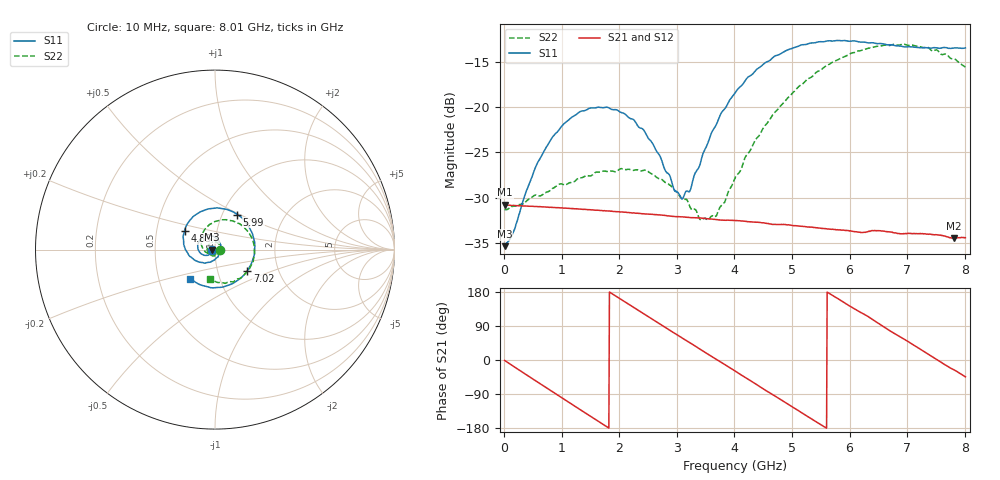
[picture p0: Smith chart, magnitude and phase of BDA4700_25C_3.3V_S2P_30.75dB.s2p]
!Agilent Technologies,E5071B,MY42404982,A.09.10
!Date: Mon Oct 20 18:16:00 2025
!Data & Calibration Information:
!Freq	S11:SOLT2(ON)	S21:SOLT2(ON)	S12:SOLT2(ON)	S22:SOLT2(ON)
# Hz S RI R 50
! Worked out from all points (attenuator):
!   801 points, 10 MHz to 8.01 GHz, reference 50 ohm
!   highest |S21| = -30.79 dB at 20 MHz (marker M1); lowest = -34.5 dB at 7.81 GHz (marker M2)
!   lowest |S11| = -35.4 dB at 10 MHz (marker M3), VSWR 1.03, Z = 48.3 - j0.0984 ohm
!   |S11| at or under -10 dB: start of sweep to end of sweep
!   |S22| runs from -32.5 to -13.0 dB; largest |S21 - S12| = 0.00036
!   S11 on the Smith chart (normalised r, x): 10 MHz: 0.97, -0.00; 4.83 GHz: 0.70, +0.15; 5.99 GHz: 1.17, +0.48; 7.02 GHz: 1.39, -0.35; 8.01 GHz: 0.72, -0.25
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1e7  -0.017 -0.00102  0.0289 -0.00063  0.0288 -0.000637  0.0272 -0.000751
2e7  -0.0174 -0.00161  0.0289 -0.00107  0.0288 -0.00118  0.0271 -0.00109
1.6e8  -0.0178 -0.00977  0.0275 -0.00803  0.0275 -0.00802  0.0273 -0.00773
5.3e8  -0.0346 -0.029  0.017 -0.0226  0.017 -0.0226  0.0168 -0.028
7.3e8  -0.0502 -0.0326  0.0083 -0.0268  0.00832 -0.0268  0.00416 -0.0336
1.35e9  -0.0952 0.00416  -0.0189 -0.0197  -0.0189 -0.0198  -0.0364 -0.0183
2.08e9  -0.0538 0.0752  -0.0239 0.011  -0.0239 0.0111  -0.0303 0.0336
2.68e9  0.0194 0.0518  -0.00323 0.0252  -0.00328 0.0252  0.0126 0.0383
2.96e9  0.032 0.0135  0.00824 0.0235  0.00817 0.0234  0.0259 0.0234
3.1e9  0.0303 -0.00763  0.0134 0.0209  0.0133 0.0209  0.0287 0.012
3.23e9  0.0234 -0.0255  0.0173 0.0174  0.0174 0.0174  0.0278 0.00306
3.55e9  -0.0142 -0.0632  0.0234 0.00605  0.0234 0.006  0.0132 -0.0199
3.69e9  -0.0381 -0.0711  0.0239 0.000541  0.024 0.00048  0.00177 -0.0252
4.01e9  -0.1008 -0.0644  0.0207 -0.0115  0.0207 -0.0114  -0.0309 -0.0259
4.83e9  -0.1698 0.1047  -0.00656 -0.0215  -0.0064 -0.0216  -0.0763 0.0707
5.35e9  -0.0735 0.2139  -0.0199 -0.00872  -0.0199 -0.00879  -0.0158 0.1467
5.99e9  0.123 0.1955  -0.0167 0.0123  -0.0168 0.0122  0.1281 0.1476
6.68e9  0.2208 -0.00762  0.00388 0.0201  0.00392 0.0201  0.2191 0.000829
7.02e9  0.1791 -0.1198  0.0134 0.015  0.0135 0.0148  0.2001 -0.0899
7.45e9  0.053 -0.2062  0.0196 0.00248  0.0197 0.00248  0.1136 -0.1701
7.81e9  -0.0758 -0.1981  0.017 -0.00824  0.017 -0.00831  0.0181 -0.1839
8.01e9  -0.1369 -0.1625  0.0136 -0.0133  0.0136 -0.0132  -0.0295 -0.1635
